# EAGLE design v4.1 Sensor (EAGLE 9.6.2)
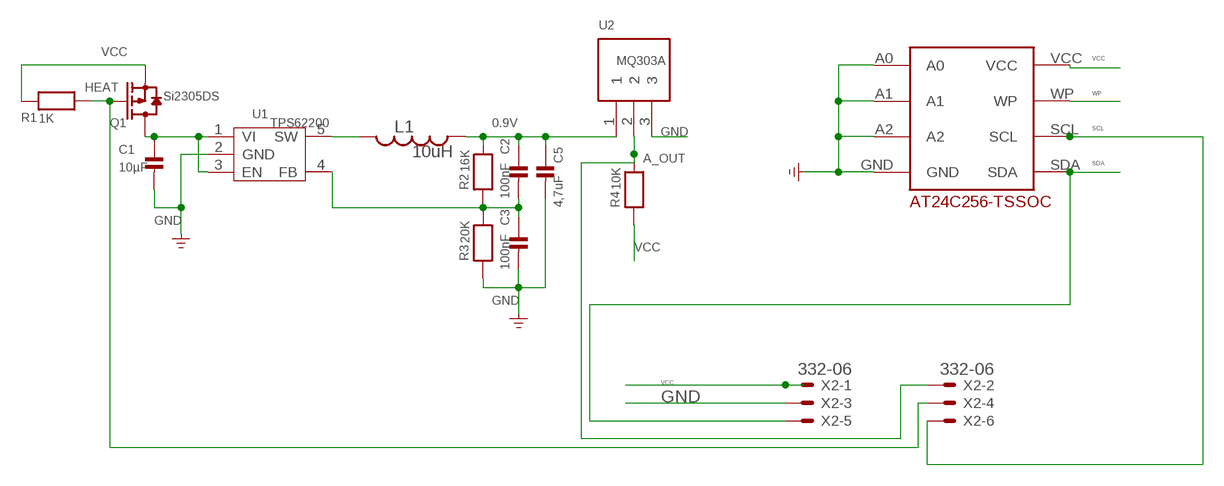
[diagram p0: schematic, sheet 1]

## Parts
C1  10µF  CAP_CERAMIC0805  [0805]
C2  100nF  CAP_CERAMIC0805  [0805]
C3  100nF  CAP_CERAMIC0805  [0805]
C5  4,7uF  CAP_CERAMIC0805  [0805]
L1  10uH  INDUCTORINCUCTOR_SENSOR  [SDR7045-100M]
Q1  Si2305DS  MOSFET-P'SI2323CDS/SI2305DS<BR>'  [SOT23]
R1  1K  RESISTOR0805  [0805]
R2  16K  RESISTOR0805  [0805]
R3  20K  RESISTOR0805  [0805]
R4  10K  RESISTOR0805  [0805]
U1  TPS62200  TPS62200DBV  [SOT23-5]
U2  MQ303A  [MQ303A]
U$1  DECADE-AT24C256-10TI-2.7  [DECADE-AT24CXX]
X2  332-06  [332-06]

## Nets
0.9V: C2.1 C5.1 L1.1 R2.2 U2.1
A_OUT: R4.2 U2.2 X2.2
GND: C1.2 C3.2 C5.2 R3.1 U1.2(GND) U2.3 U$1.A0 U$1.A1 U$1.A2 U$1.GND X2.3
HEAT: Q1.1(G) R1.2 X2.4
N$1: C1.1 Q1.3(D) U1.1(VI) U1.3(EN)
N$2: L1.2 U1.5(SW)
N$3: C2.2 C3.1 R2.1 R3.2 U1.4(FB)
SCL: U$1.SCL X2.6
SDA: U$1.SDA X2.5
VCC: Q1.2(S) R1.1 R4.1 U$1.VCC X2.1
WP: U$1.WP

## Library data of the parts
C1 = microbuilder:CAP_CERAMIC: Ceramic Capacitors; MPN: GRM21BR71A106KA73K
C2 C3 = microbuilder:CAP_CERAMIC: Ceramic Capacitors; MPN: C0805C104K8RACAUTO
C5 = microbuilder:CAP_CERAMIC: Ceramic Capacitors; MPN: 0805ZG475ZAT4A
L1 = passives:INDUCTOR: A very specific inductor
Q1 = discrete:MOSFET-P; MPN: SI2305DS
R1 = microbuilder:RESISTOR: Resistors; MPN: RP73PF2A1K0BTDF
R2 = microbuilder:RESISTOR: Resistors; MPN: RK73H2ARTTD1602F
R3 = microbuilder:RESISTOR: Resistors; MPN: RCC080520K0FKEA
R4 = microbuilder:RESISTOR: Resistors; MPN: RCC080510K0FKEA
U1 = IC:TPS62200: High-Efficiency,SOT23 STEP-DOWN,DC-DC Converter; MPN: TPS62200DBVR
U2 = MQ303A:MQ303A; MPN: MQ303B
U$1 = DECADE-libraries20151104:DECADE-AT24C256-10TI-2.7; MPN: AT24C256-TSSOC
X2 = con-garry:332-06: 6 Pin - 2mm Dual Row Source: www.mpe-connector.de / garry_shortform_2012.pdf; MPN: 6 Pin - 2mm Dual Row

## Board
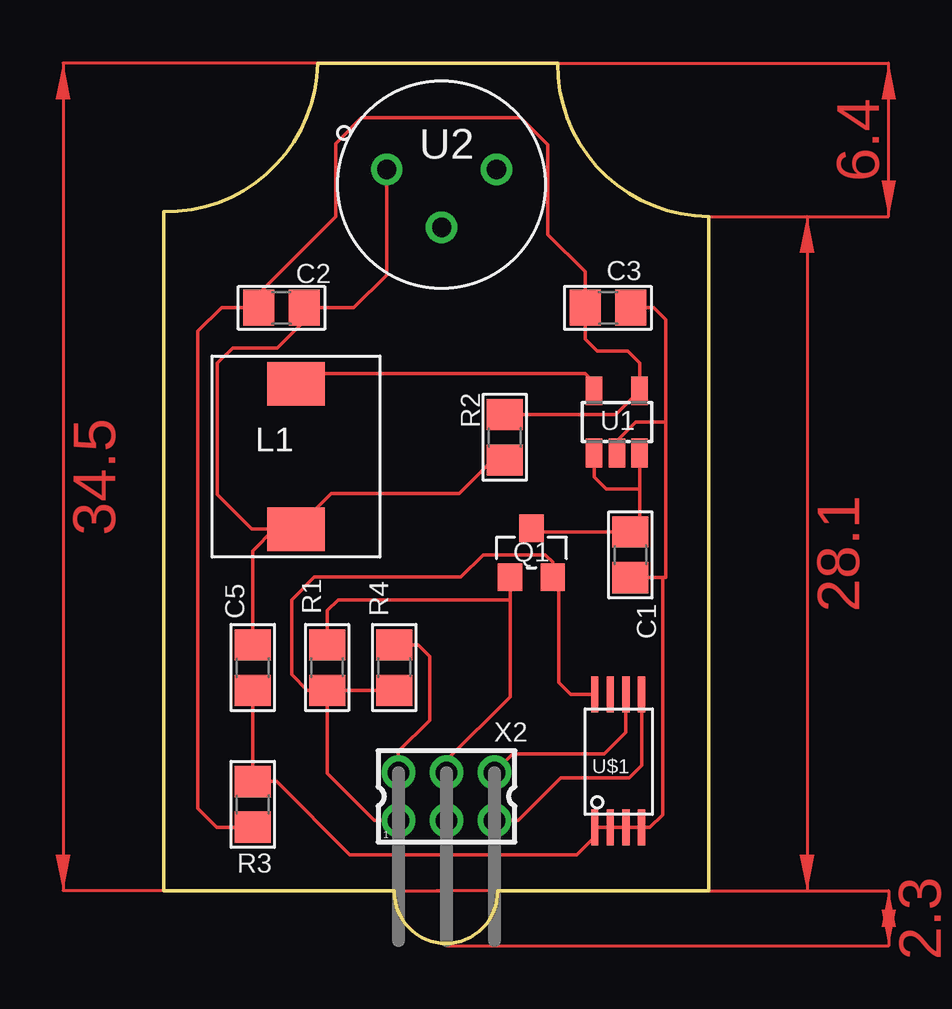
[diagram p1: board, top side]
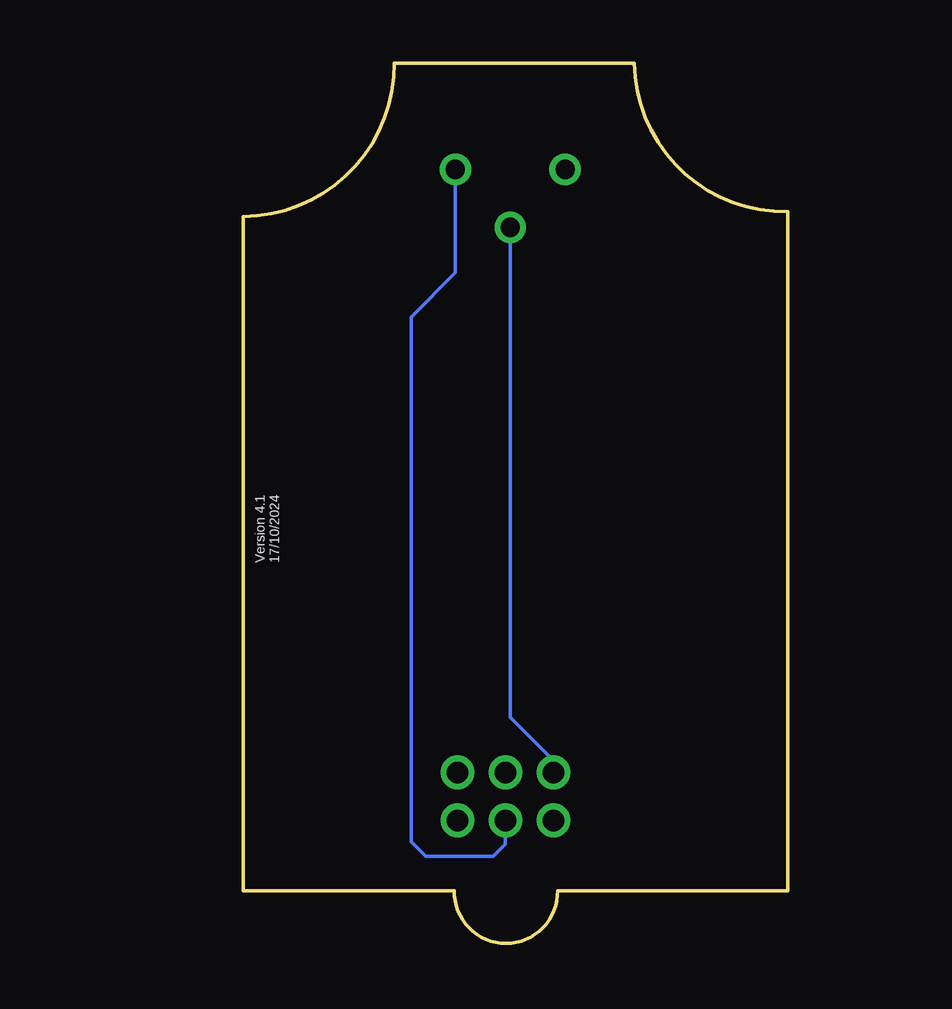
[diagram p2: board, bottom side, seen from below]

Size 22.7 x 36.7 mm. Coordinates in mm from the lower left corner, seen from the top.
Outline: 0,30.5 0,2.2 9.6,2.2 arc183 13.9,2.2 22.7,2.2 22.7,30.3 arc-90 16.4,36.7 6.4,36.7 arc-90 0,30.5
Copper layers (1*16): Top 0.035mm / dielectric 1.5mm / Bottom 0.035mm
Design rules "default": minimum track width 6mil, minimum drill 0.35mm, track to track 6mil, track to pad 6mil, pad to pad 6mil, via to via 6mil, smd to smd 6mil, copper to edge 40mil, drill to drill 6mil, minimum pad ring 10mil, minimum via ring 8mil, stop-mask expansion 4mil, vias tented up to drill 0mil, thermal gap 10mil

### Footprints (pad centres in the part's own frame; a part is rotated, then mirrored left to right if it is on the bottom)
0805 = smd 1.3 x 1.5: 1 -0.95,0; 2 0.95,0
SDR7045-100M = smd 1.8 x 2.4: 1 -3.031,0; 2 3.031,0
SOT23 = smd 1.016 x 1.143: 1 -0.889,-1.016; 2 0.889,-1.016; 3 0,1.016
SOT23-5 = smd 0.69 x 1.2: 1 -0.95,-1.3; 2 0,-1.3; 3 0.95,-1.3; 4 0.95,1.3; 5 -0.95,1.3
MQ303A = drill 0.8: 1 -2.286,0.635; 2 0,-1.778; 3 2.286,0.635
DECADE-AT24CXX = smd 1.5 x 0.3: A0 -2.75,1; A1 -2.75,0.35; A2 -2.75,-0.3; GND -2.75,-0.95; SCL 2.8,-0.3; SDA 2.8,-0.95; VCC 2.8,1; WP 2.8,0.35
332-06 = drill 0.9 pad 1.27: 1 -2,-1; 2 -2,1; 3 0,-1; 4 0,1; 5 2,-1; 6 2,1

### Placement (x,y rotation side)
C1  19.43,16.2 270 top
C2  4.9,26.5 180 top
C3  18.5,26.5 0 top
C5  3.7,11.5 270 top
L1  5.5,20.3 90 top
Q1  15.31,16.29 0 top
R1  6.8,11.5 90 top
R2  14.2,21.1 270 top
R3  3.7,5.8 270 top
R4  9.6,11.5 90 top
U1  18.87,21.74 0 top
U2  11.57,31.63 0 top
U$1  18.95,7.58 90 top
X2  11.77,6.13 0 top

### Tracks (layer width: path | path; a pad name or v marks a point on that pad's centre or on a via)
0.9V
  Top 0.152: 6.4,26.5 7.92,26.5 9.28,27.87 U2.1 | 6.4,26.5 C2.1 | 6.4,26.5 4.73,24.83 2.86,24.83 2.23,24.2 2.23,18.71 3.67,17.27 L1.1 | R2.2 13.7,20.15 12.3,18.75 6.98,18.75 L1.1 | C5.1 3.7,16.37 4.6,17.27 L1.1
A_OUT
  Top 0.152: X2.2 9.77,8 11.08,9.31 11.08,11.97 10.6,12.45 R4.2
  Bottom 0.152: U2.2 11.57,9.43 9.77,7.63 X2.2
GND
  Top 0.152: 20.91,21.74 19.67,21.74 18.87,20.94 U1.2 | 20.91,21.74 20.91,15.25 C1.2 20.78,15.25 20.78,5.37 20.24,4.83 U$1.GND U$1.A2 U$1.A1 U$1.A0 17.95,4.45 17.2,3.7 11.77,3.7 X2.3 11.77,3.81 11.66,3.7 7.75,3.7 4.7,6.75 R3.1 C5.2 | 20.91,21.74 20.91,26 20.41,26.5 C3.2
  Bottom 0.152: U2.3 13.86,27.97 15.7,26.12 15.7,4.24 15.09,3.63 12.27,3.63 11.77,4.13 X2.3
HEAT
  Top 0.152: R1.2 6.8,13.87 7.25,14.33 14.42,14.33 | X2.4 11.77,7.62 14.42,10.27 14.42,14.33 | 14.42,14.33 Q1.1
N$1
  Top 0.152: Q1.3 15.47,17.15 C1.1 19.82,17.54 19.82,18.94 | 19.82,18.94 18.42,18.94 17.92,19.44 U1.1 | U1.3 19.82,18.94
N$2
  Top 0.152: U1.5 17.92,23.39 17.55,23.76 7.4,23.76 7.3,23.76 5.93,23.76 L1.2
N$3
  Top 0.152: R2.1 18.82,22.04 U1.4 19.82,24.2 19.32,24.7 18.05,24.7 17.55,25.2 C3.1 17.55,28 16,29.55 16,33.3 14.87,34.43 8.23,34.43 7.15,33.34 7.15,30.3 3.95,27.1 C2.2 2.4,26.5 1.42,25.52 1.42,5.63 2.2,4.85 R3.2
SCL
  Top 0.152: U$1.SCL 19.25,8.81 18.34,7.9 14.54,7.9 X2.6
SDA
  Top 0.152: X2.5 14.77,5.13 16.54,6.9 19.38,6.9 19.9,7.42 U$1.SDA
VCC
  Top 0.152: X2.1 8.77,5.13 6.8,7.1 R1.1 | R1.1 R4.1 | U$1.VCC 16.95,10.38 16.45,10.88 16.45,15.02 Q1.2 16.2,15.9 15.9,16.2 13.3,16.2 12.37,15.27 6.27,15.27 5.32,14.33 5.32,11.21 5.98,10.55 R1.1
(copper drawn outside any net)
  shapes: Top area x7

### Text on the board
bPlace: Version 4.1 / 17/10/2024
tNames: U$1

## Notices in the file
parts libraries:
DECADE-libraries20151104: Licensing: Creative Commons ShareAlike 4.0 International - https://creativecommons.org/licenses/by-sa/4.0
